(* Logix 5000 AddOnInstructionDefinition export Banner_TL70Pro_Param_v4; software revision 33.00; part 2 of 3 *)
(* tags used below, declared in another part *)
   TL70Pro : Banner_TL70Pro_v4;
   Port_Data : Banner_IOL_Port_v4;
   Port : INT;   // Port Number that device is plugged into.
   Local_Control : DINT;
   Command_Being_Processed : BOOL;
   Update_Archive : BOOL;
   Index_Write_Inprocess : DINT;
   Index_Write_Control : DINT;
   Inprocess_Index : DINT;
   BS_Index : DINT;
   Index_W : DINT;
   W_Index : DINT;
   GT_Index2 : DINT;
   GT_Index1 : DINT;
   LT_Index2 : DINT;
   LT_Index1 : DINT;
(* Banner_TL70Pro_Param_v4, continued *)

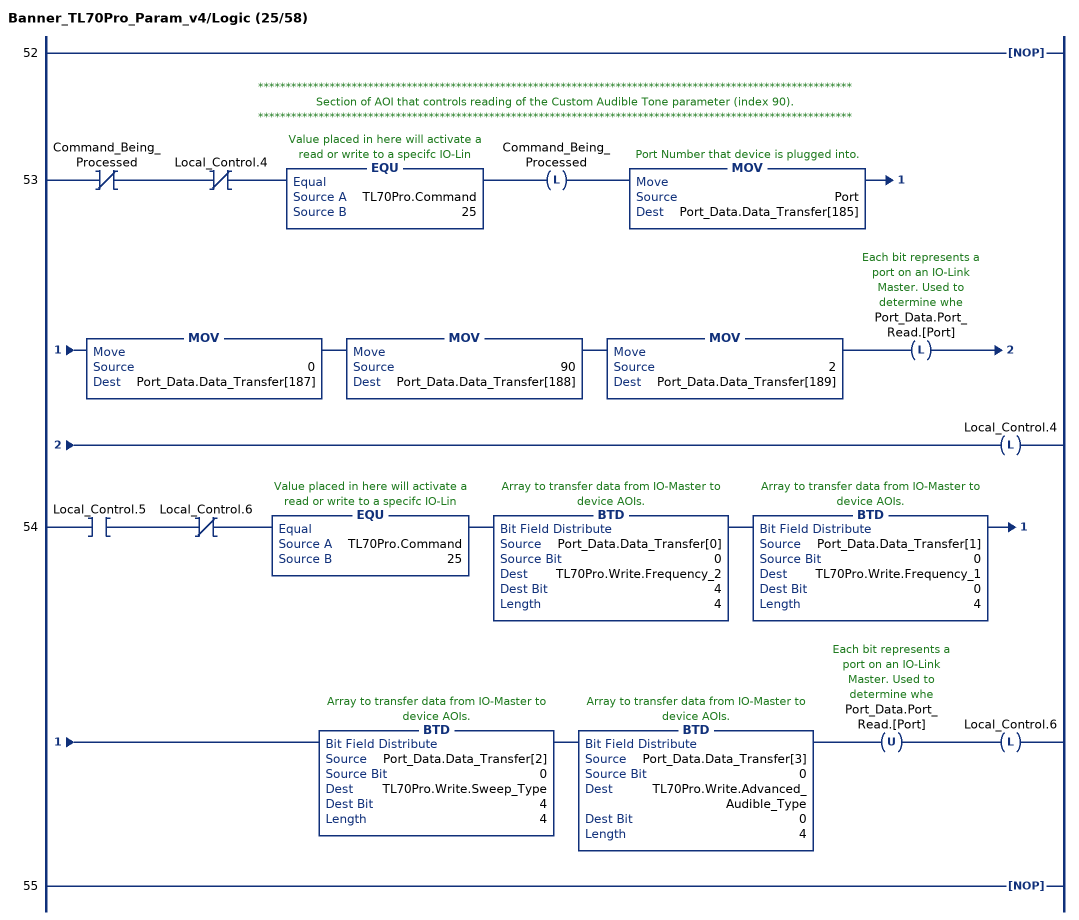
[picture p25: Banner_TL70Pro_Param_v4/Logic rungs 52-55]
   52: NOP();
   // ************************************************************************************************************
   // Section of AOI that controls reading of the Custom Audible Tone parameter (index 90).
   // ************************************************************************************************************
   53: XIO(Command_Being_Processed)XIO(Local_Control.4)EQU(TL70Pro.Command,25)OTL(Command_Being_Processed)MOV(Port,Port_Data.Data_Transfer[185])MOV(0,Port_Data.Data_Transfer[187])MOV(90,Port_Data.Data_Transfer[188])MOV(2,Port_Data.Data_Transfer[189])OTL(Port_Data.Port_Read.[Port])OTL(Local_Control.4);
   54: XIC(Local_Control.5)XIO(Local_Control.6)EQU(TL70Pro.Command,25)BTD(Port_Data.Data_Transfer[0],0,TL70Pro.Write.Frequency_2,4,4)BTD(Port_Data.Data_Transfer[1],0,TL70Pro.Write.Frequency_1,0,4)BTD(Port_Data.Data_Transfer[2],0,TL70Pro.Write.Sweep_Type,4,4)BTD(Port_Data.Data_Transfer[3],0,TL70Pro.Write.Advanced_Audible_Type,0,4)OTU(Port_Data.Port_Read.[Port])OTL(Local_Control.6);
   55: NOP();
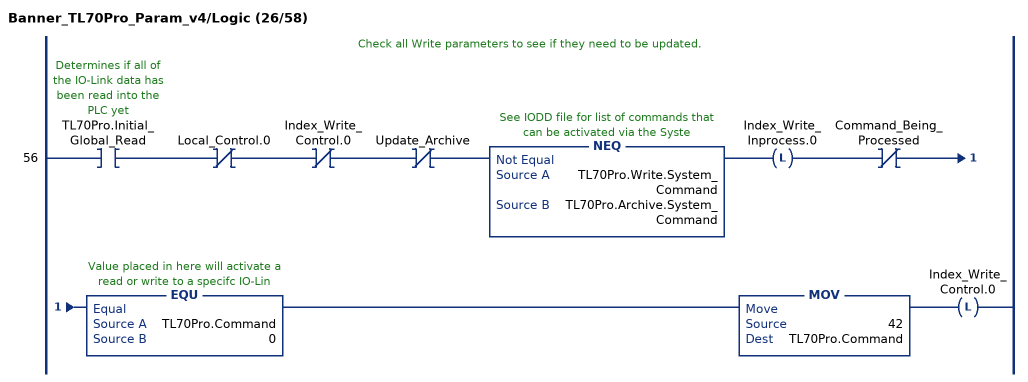
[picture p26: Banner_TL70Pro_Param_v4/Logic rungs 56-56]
   // Check all Write parameters to see if they need to be updated.
   56: XIC(TL70Pro.Initial_Global_Read)XIO(Local_Control.0)XIO(Index_Write_Control.0)XIO(Update_Archive)NEQ(TL70Pro.Write.System_Command,TL70Pro.Archive.System_Command)OTL(Index_Write_Inprocess.0)XIO(Command_Being_Processed)EQU(TL70Pro.Command,0)MOV(42,TL70Pro.Command)OTL(Index_Write_Control.0);
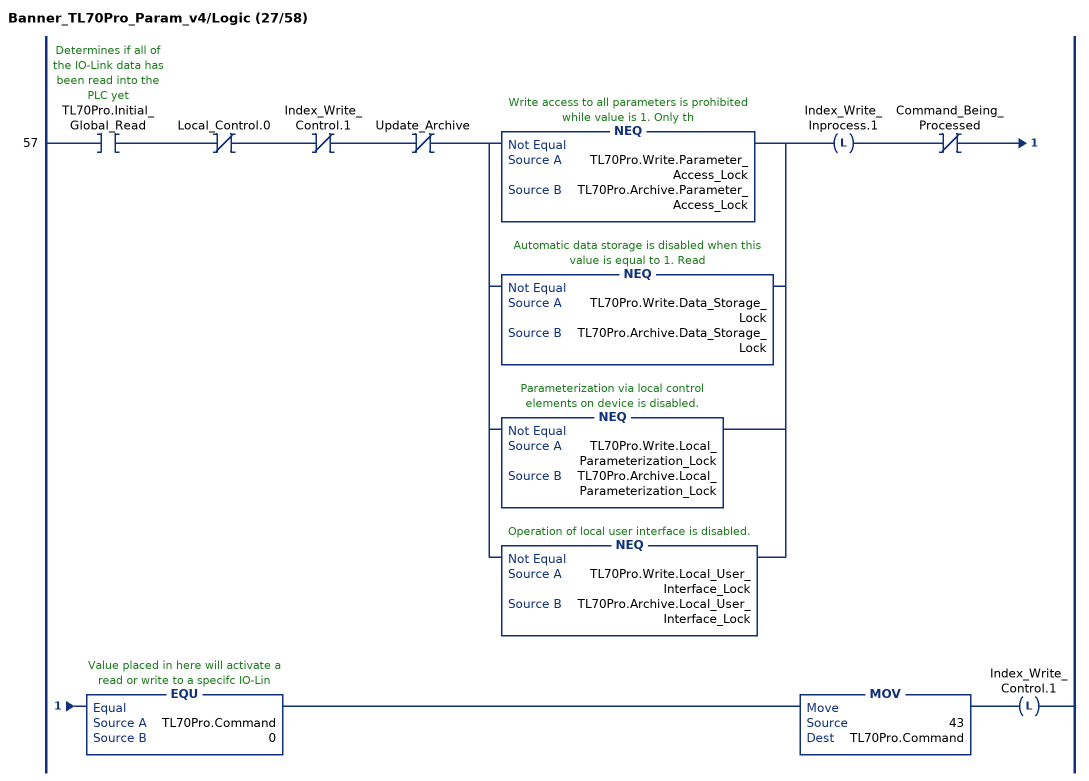
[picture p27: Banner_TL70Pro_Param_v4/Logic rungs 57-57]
   57: XIC(TL70Pro.Initial_Global_Read)XIO(Local_Control.0)XIO(Index_Write_Control.1)XIO(Update_Archive)[NEQ(TL70Pro.Write.Parameter_Access_Lock,TL70Pro.Archive.Parameter_Access_Lock) ,NEQ(TL70Pro.Write.Data_Storage_Lock,TL70Pro.Archive.Data_Storage_Lock) ,NEQ(TL70Pro.Write.Local_Parameterization_Lock,TL70Pro.Archive.Local_Parameterization_Lock) ,NEQ(TL70Pro.Write.Local_User_Interface_Lock,TL70Pro.Archive.Local_User_Interface_Lock) ]OTL(Index_Write_Inprocess.1)XIO(Command_Being_Processed)EQU(TL70Pro.Command,0)MOV(43,TL70Pro.Command)OTL(Index_Write_Control.1);
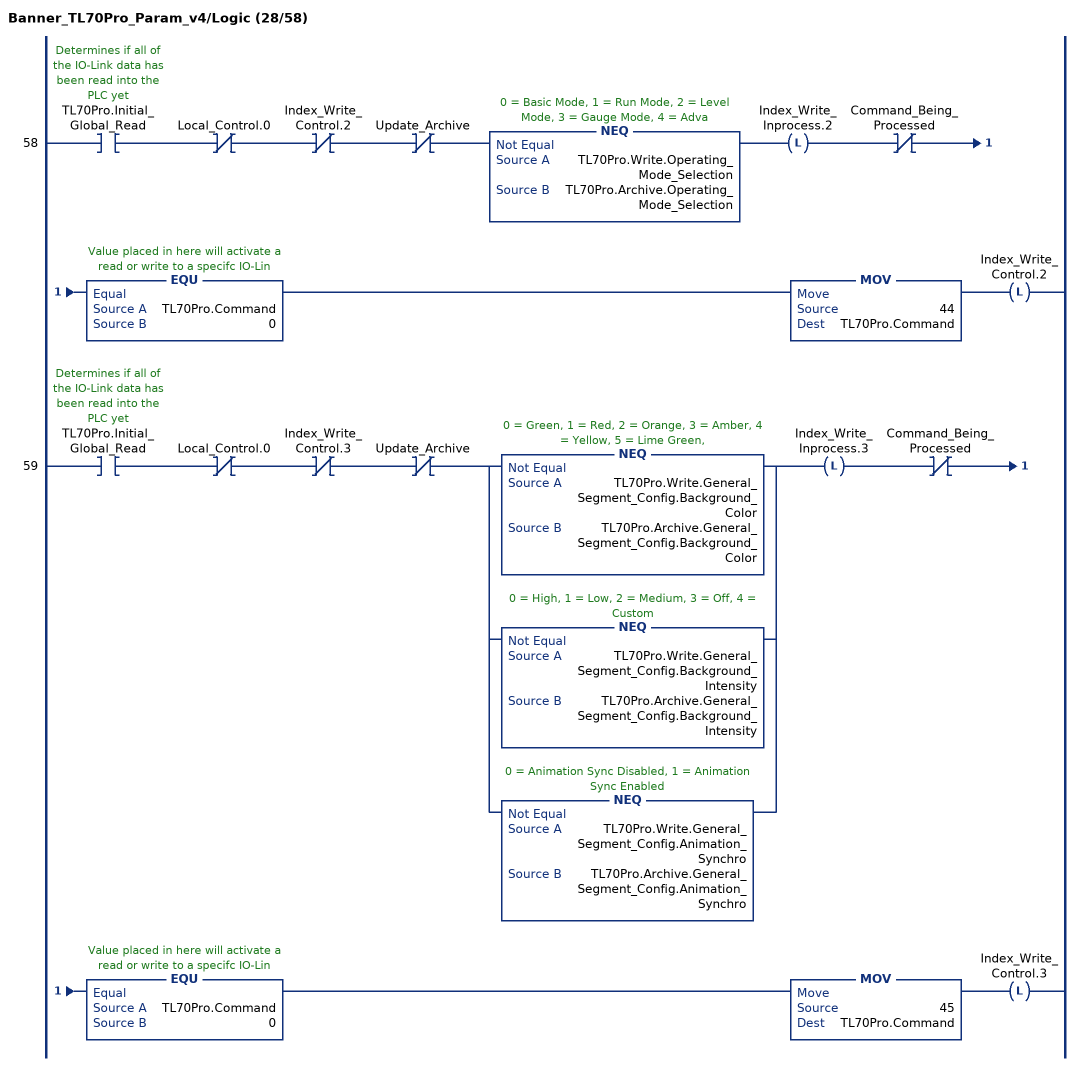
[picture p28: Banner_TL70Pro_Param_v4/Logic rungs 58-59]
   58: XIC(TL70Pro.Initial_Global_Read)XIO(Local_Control.0)XIO(Index_Write_Control.2)XIO(Update_Archive)NEQ(TL70Pro.Write.Operating_Mode_Selection,TL70Pro.Archive.Operating_Mode_Selection)OTL(Index_Write_Inprocess.2)XIO(Command_Being_Processed)EQU(TL70Pro.Command,0)MOV(44,TL70Pro.Command)OTL(Index_Write_Control.2);
   59: XIC(TL70Pro.Initial_Global_Read)XIO(Local_Control.0)XIO(Index_Write_Control.3)XIO(Update_Archive)[NEQ(TL70Pro.Write.General_Segment_Config.Background_Color,TL70Pro.Archive.General_Segment_Config.Background_Color) ,NEQ(TL70Pro.Write.General_Segment_Config.Background_Intensity,TL70Pro.Archive.General_Segment_Config.Background_Intensity) ,NEQ(TL70Pro.Write.General_Segment_Config.Animation_Synchro,TL70Pro.Archive.General_Segment_Config.Animation_Synchro) ]OTL(Index_Write_Inprocess.3)XIO(Command_Being_Processed)EQU(TL70Pro.Command,0)MOV(45,TL70Pro.Command)OTL(Index_Write_Control.3);
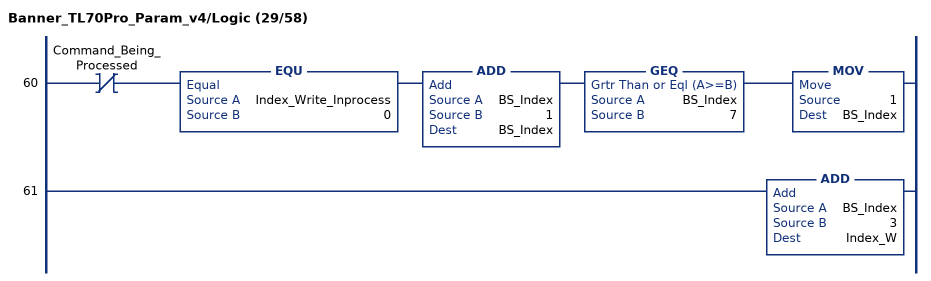
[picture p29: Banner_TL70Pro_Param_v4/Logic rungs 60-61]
   60: XIO(Command_Being_Processed)EQU(Index_Write_Inprocess,0)ADD(BS_Index,1,BS_Index)GEQ(BS_Index,7)MOV(1,BS_Index);
   61: ADD(BS_Index,3,Index_W);
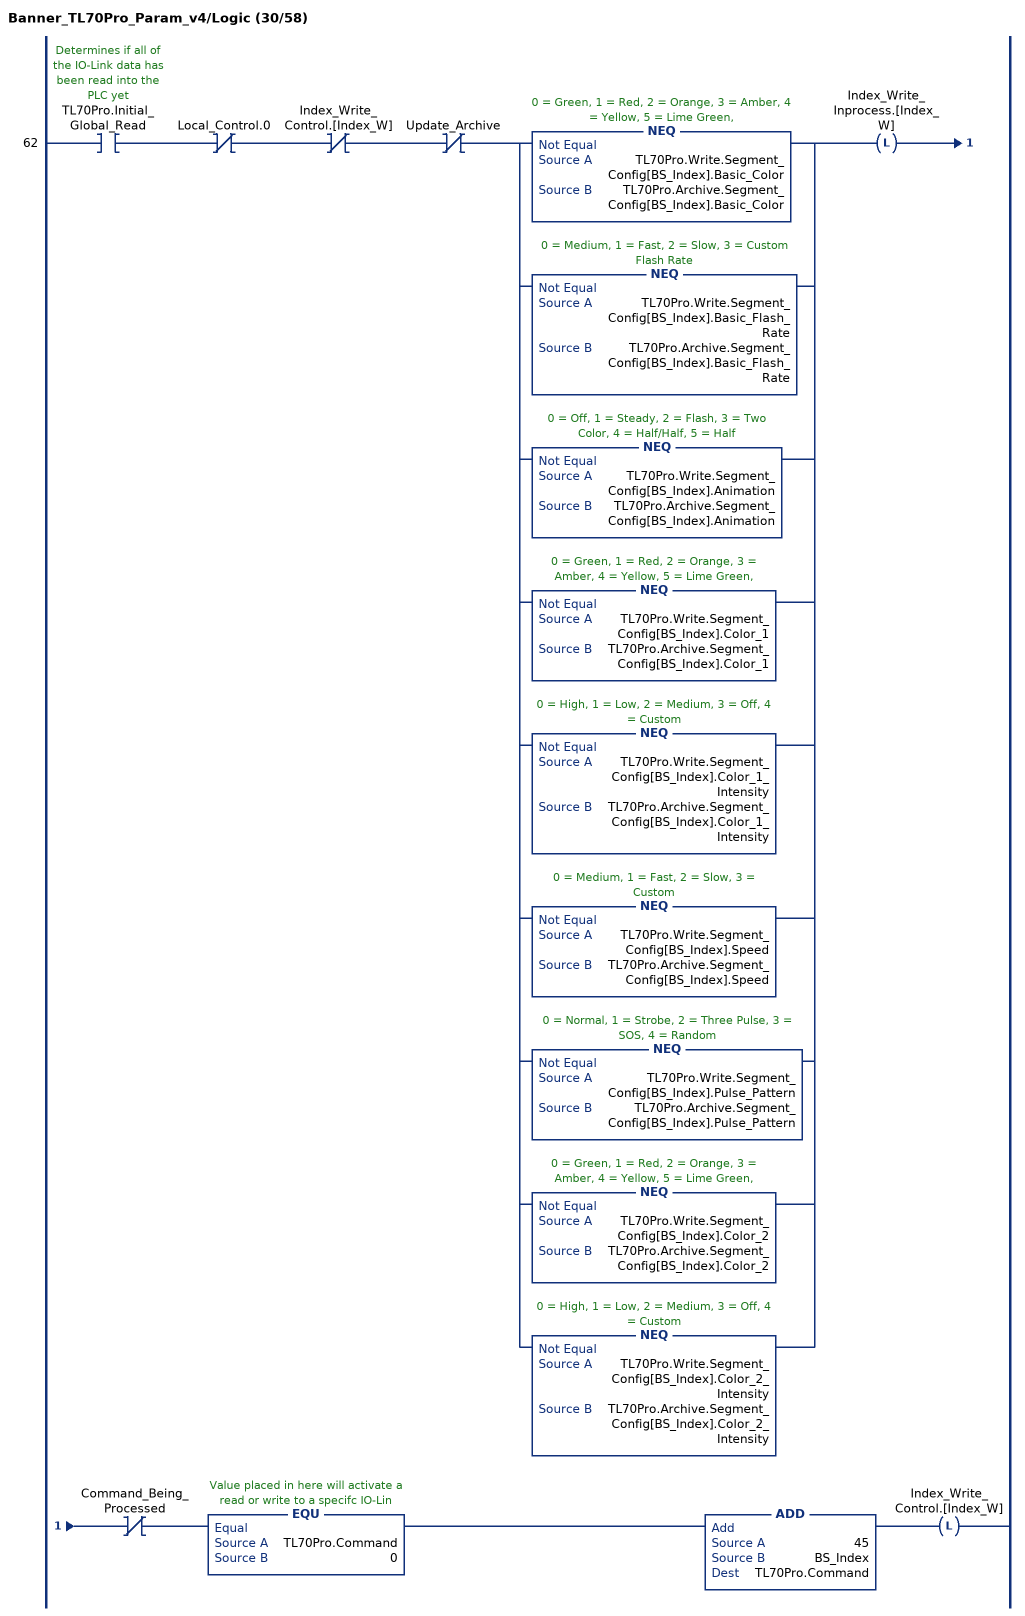
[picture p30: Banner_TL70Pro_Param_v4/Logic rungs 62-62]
   62: XIC(TL70Pro.Initial_Global_Read)XIO(Local_Control.0)XIO(Index_Write_Control.[Index_W])XIO(Update_Archive)[NEQ(TL70Pro.Write.Segment_Config[BS_Index].Basic_Color,TL70Pro.Archive.Segment_Config[BS_Index].Basic_Color) ,NEQ(TL70Pro.Write.Segment_Config[BS_Index].Basic_Flash_Rate,TL70Pro.Archive.Segment_Config[BS_Index].Basic_Flash_Rate) ,NEQ(TL70Pro.Write.Segment_Config[BS_Index].Animation,TL70Pro.Archive.Segment_Config[BS_Index].Animation) ,NEQ(TL70Pro.Write.Segment_Config[BS_Index].Color_1,TL70Pro.Archive.Segment_Config[BS_Index].Color_1) ,NEQ(TL70Pro.Write.Segment_Config[BS_Index].Color_1_Intensity,TL70Pro.Archive.Segment_Config[BS_Index].Color_1_Intensity) ,NEQ(TL70Pro.Write.Segment_Config[BS_Index].Speed,TL70Pro.Archive.Segment_Config[BS_Index].Speed) ,NEQ(TL70Pro.Write.Segment_Config[BS_Index].Pulse_Pattern,TL70Pro.Archive.Segment_Config[BS_Index].Pulse_Pattern) ,NEQ(TL70Pro.Write.Segment_Config[BS_Index].Color_2,TL70Pro.Archive.Segment_Config[BS_Index].Color_2) ,NEQ(TL70Pro.Write.Segment_Config[BS_Index].Color_2_Intensity,TL70Pro.Archive.Segment_Config[BS_Index].Color_2_Intensity) ]OTL(Index_Write_Inprocess.[Index_W])XIO(Command_Being_Processed)EQU(TL70Pro.Command,0)ADD(45,BS_Index,TL70Pro.Command)OTL(Index_Write_Control.[Index_W]);
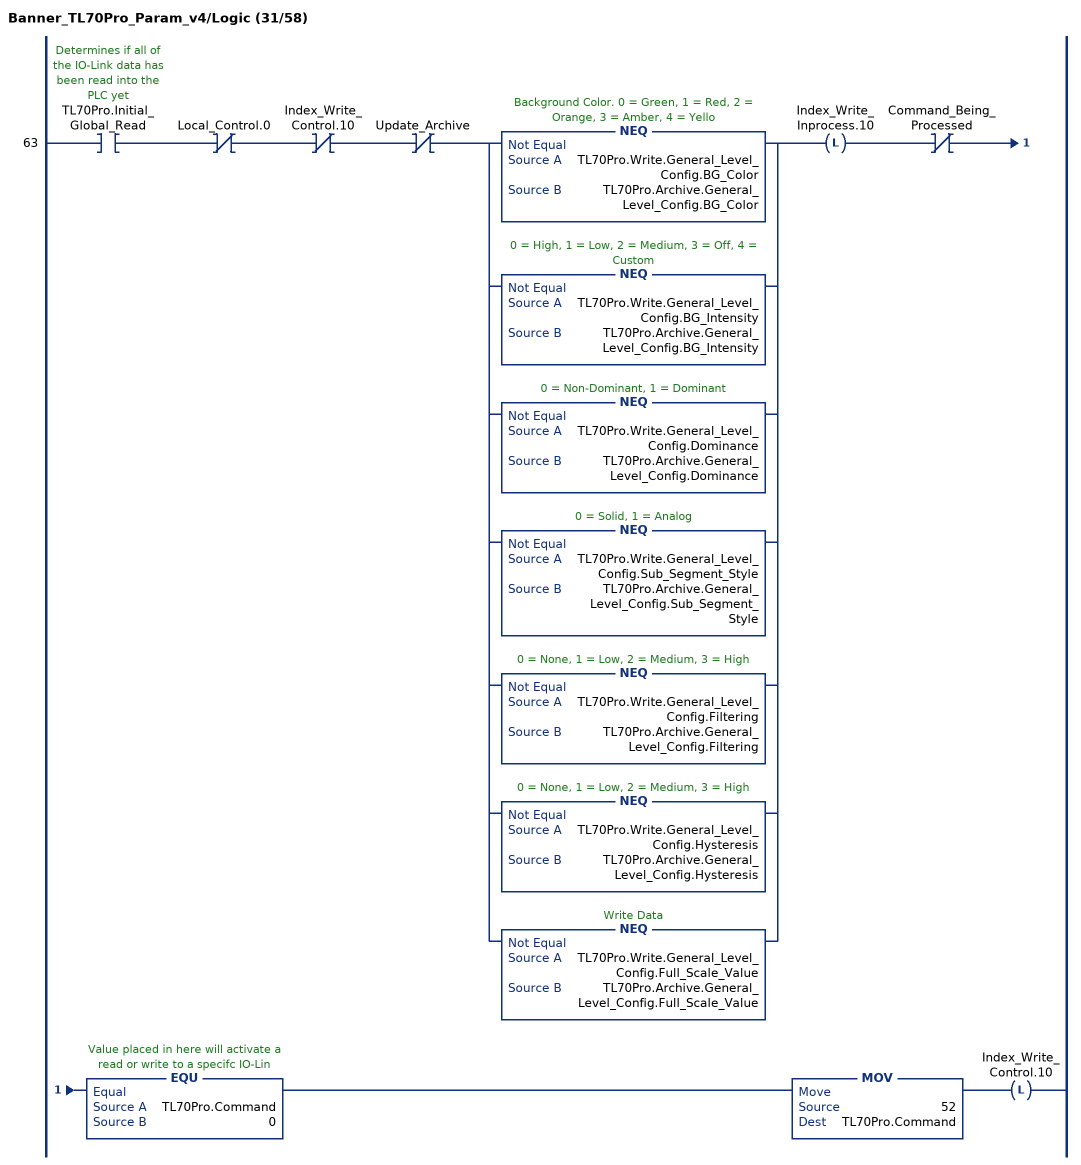
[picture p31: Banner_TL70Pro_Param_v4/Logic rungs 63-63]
   63: XIC(TL70Pro.Initial_Global_Read)XIO(Local_Control.0)XIO(Index_Write_Control.10)XIO(Update_Archive)[NEQ(TL70Pro.Write.General_Level_Config.BG_Color,TL70Pro.Archive.General_Level_Config.BG_Color) ,NEQ(TL70Pro.Write.General_Level_Config.BG_Intensity,TL70Pro.Archive.General_Level_Config.BG_Intensity) ,NEQ(TL70Pro.Write.General_Level_Config.Dominance,TL70Pro.Archive.General_Level_Config.Dominance) ,NEQ(TL70Pro.Write.General_Level_Config.Sub_Segment_Style,TL70Pro.Archive.General_Level_Config.Sub_Segment_Style) ,NEQ(TL70Pro.Write.General_Level_Config.Filtering,TL70Pro.Archive.General_Level_Config.Filtering) ,NEQ(TL70Pro.Write.General_Level_Config.Hysteresis,TL70Pro.Archive.General_Level_Config.Hysteresis) ,NEQ(TL70Pro.Write.General_Level_Config.Full_Scale_Value,TL70Pro.Archive.General_Level_Config.Full_Scale_Value) ]OTL(Index_Write_Inprocess.10)XIO(Command_Being_Processed)EQU(TL70Pro.Command,0)MOV(52,TL70Pro.Command)OTL(Index_Write_Control.10);
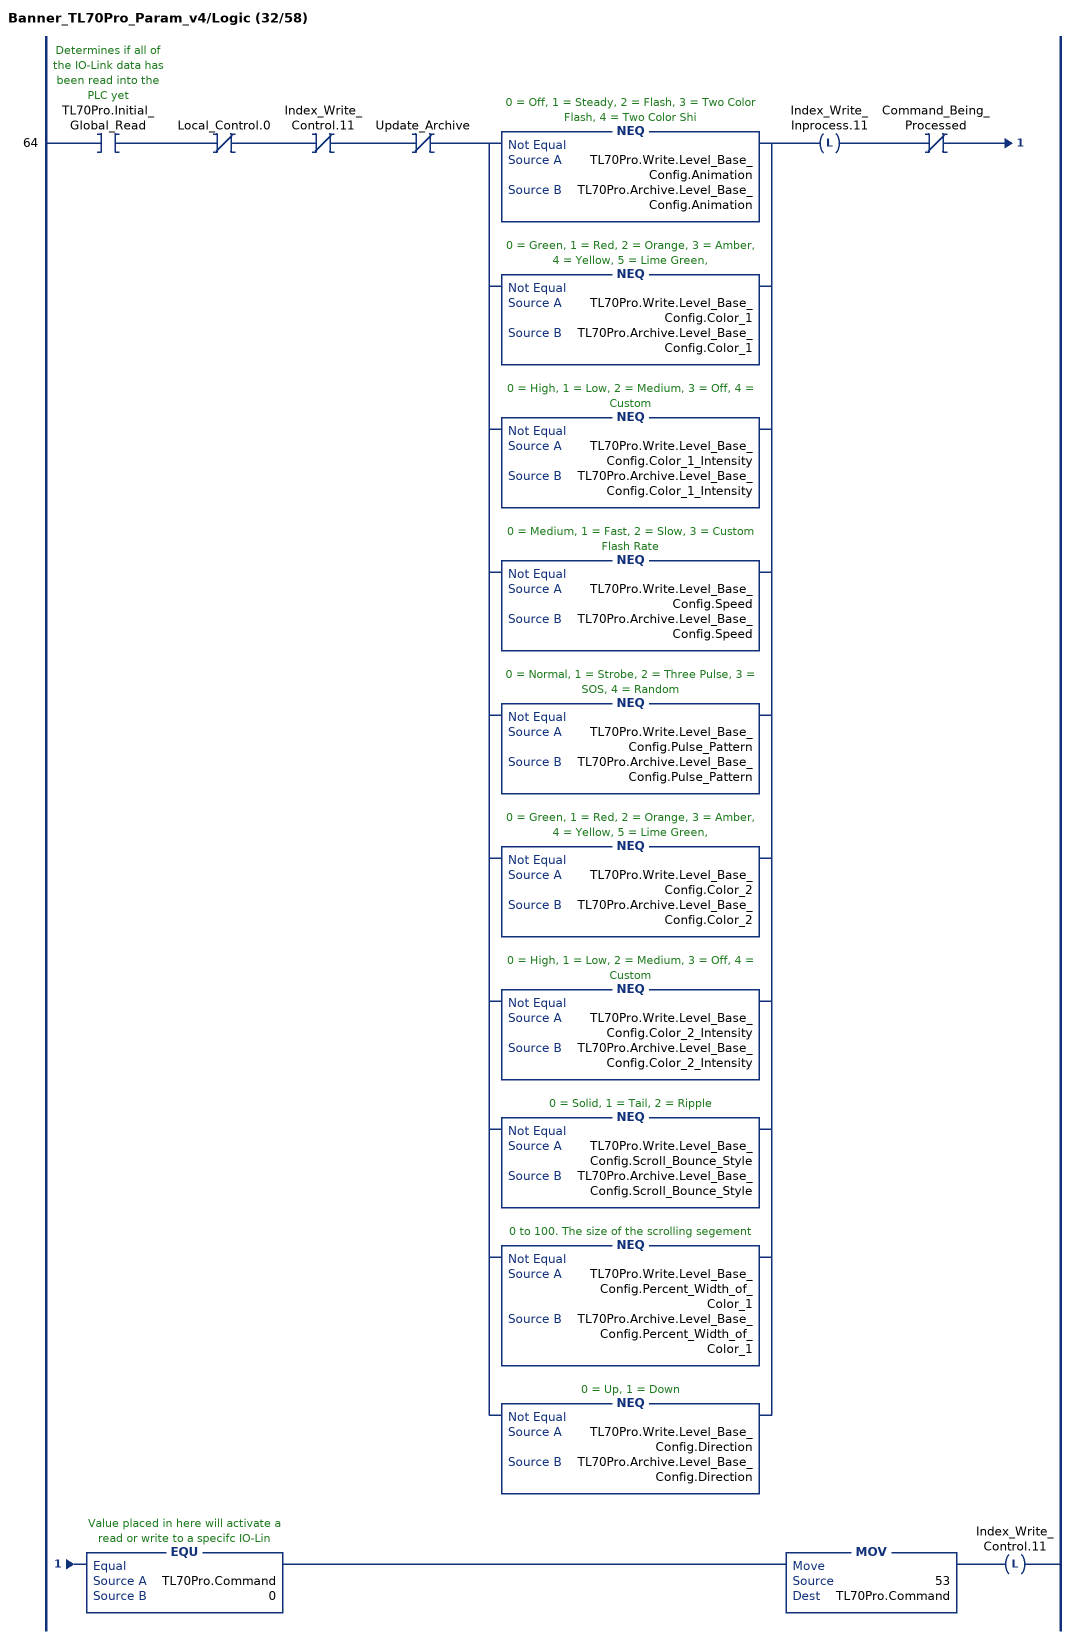
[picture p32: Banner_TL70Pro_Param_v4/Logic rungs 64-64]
   64: XIC(TL70Pro.Initial_Global_Read)XIO(Local_Control.0)XIO(Index_Write_Control.11)XIO(Update_Archive)[NEQ(TL70Pro.Write.Level_Base_Config.Animation,TL70Pro.Archive.Level_Base_Config.Animation) ,NEQ(TL70Pro.Write.Level_Base_Config.Color_1,TL70Pro.Archive.Level_Base_Config.Color_1) ,NEQ(TL70Pro.Write.Level_Base_Config.Color_1_Intensity,TL70Pro.Archive.Level_Base_Config.Color_1_Intensity) ,NEQ(TL70Pro.Write.Level_Base_Config.Speed,TL70Pro.Archive.Level_Base_Config.Speed) ,NEQ(TL70Pro.Write.Level_Base_Config.Pulse_Pattern,TL70Pro.Archive.Level_Base_Config.Pulse_Pattern) ,NEQ(TL70Pro.Write.Level_Base_Config.Color_2,TL70Pro.Archive.Level_Base_Config.Color_2) ,NEQ(TL70Pro.Write.Level_Base_Config.Color_2_Intensity,TL70Pro.Archive.Level_Base_Config.Color_2_Intensity) ,NEQ(TL70Pro.Write.Level_Base_Config.Scroll_Bounce_Style,TL70Pro.Archive.Level_Base_Config.Scroll_Bounce_Style) ,NEQ(TL70Pro.Write.Level_Base_Config.Percent_Width_of_Color_1,TL70Pro.Archive.Level_Base_Config.Percent_Width_of_Color_1) ,NEQ(TL70Pro.Write.Level_Base_Config.Direction,TL70Pro.Archive.Level_Base_Config.Direction) ]OTL(Index_Write_Inprocess.11)XIO(Command_Being_Processed)EQU(TL70Pro.Command,0)MOV(53,TL70Pro.Command)OTL(Index_Write_Control.11);
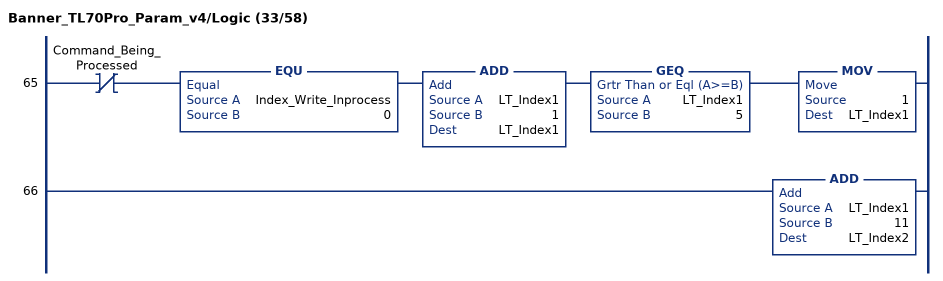
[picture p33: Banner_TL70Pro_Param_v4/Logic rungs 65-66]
   65: XIO(Command_Being_Processed)EQU(Index_Write_Inprocess,0)ADD(LT_Index1,1,LT_Index1)GEQ(LT_Index1,5)MOV(1,LT_Index1);
   66: ADD(LT_Index1,11,LT_Index2);
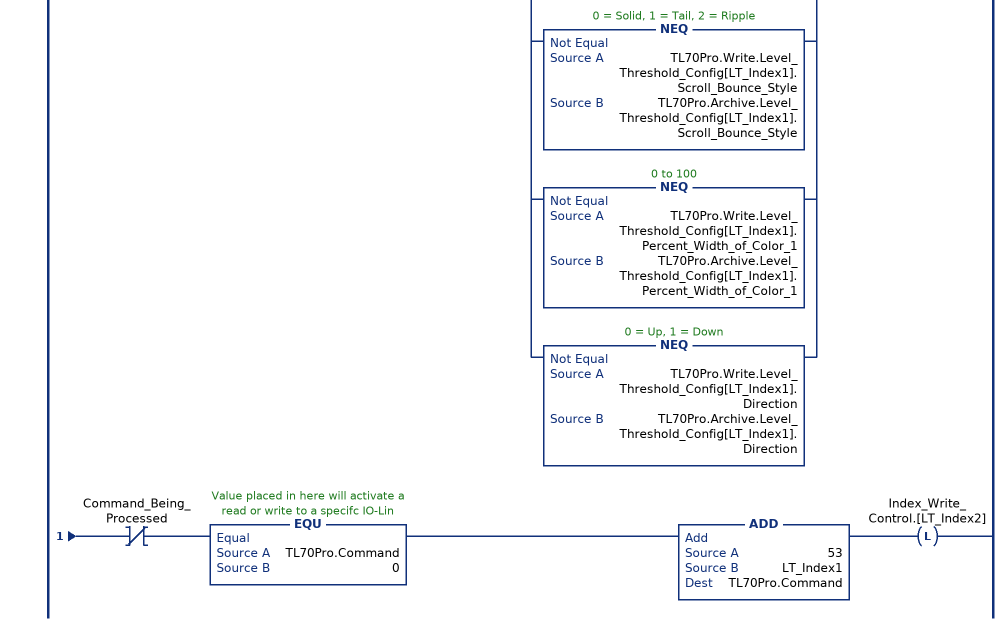
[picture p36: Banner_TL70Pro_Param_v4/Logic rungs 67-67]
   67: XIC(TL70Pro.Initial_Global_Read)XIO(Local_Control.0)XIO(Index_Write_Control.[LT_Index2])XIO(Update_Archive)[NEQ(TL70Pro.Write.Level_Threshold_Config[LT_Index1].Threshold_Enable,TL70Pro.Archive.Level_Threshold_Config[LT_Index1].Threshold_Enable) ,NEQ(TL70Pro.Write.Level_Threshold_Config[LT_Index1].Threshold_Value_Percent,TL70Pro.Archive.Level_Threshold_Config[LT_Index1].Threshold_Value_Percent) ,NEQ(TL70Pro.Write.Level_Threshold_Config[LT_Index1].Threshold_Comparison,TL70Pro.Archive.Level_Threshold_Config[LT_Index1].Threshold_Comparison) ,NEQ(TL70Pro.Write.Level_Threshold_Config[LT_Index1].Threshold_Override,TL70Pro.Archive.Level_Threshold_Config[LT_Index1].Threshold_Override) ,NEQ(TL70Pro.Write.Level_Threshold_Config[LT_Index1].Animation,TL70Pro.Archive.Level_Threshold_Config[LT_Index1].Animation) ,NEQ(TL70Pro.Write.Level_Threshold_Config[LT_Index1].Color_1,TL70Pro.Archive.Level_Threshold_Config[LT_Index1].Color_1) ,NEQ(TL70Pro.Write.Level_Threshold_Config[LT_Index1].Color_1_Intensity,TL70Pro.Archive.Level_Threshold_Config[LT_Index1].Color_1_Intensity) ,NEQ(TL70Pro.Write.Level_Threshold_Config[LT_Index1].Speed,TL70Pro.Archive.Level_Threshold_Config[LT_Index1].Speed) ,NEQ(TL70Pro.Write.Level_Threshold_Config[LT_Index1].Pulse_Pattern,TL70Pro.Archive.Level_Threshold_Config[LT_Index1].Pulse_Pattern) ,NEQ(TL70Pro.Write.Level_Threshold_Config[LT_Index1].Color_2,TL70Pro.Archive.Level_Threshold_Config[LT_Index1].Color_2) ,NEQ(TL70Pro.Write.Level_Threshold_Config[LT_Index1].Color_2_Intensity,TL70Pro.Archive.Level_Threshold_Config[LT_Index1].Color_2_Intensity) ,NEQ(TL70Pro.Write.Level_Threshold_Config[LT_Index1].Scroll_Bounce_Style,TL70Pro.Archive.Level_Threshold_Config[LT_Index1].Scroll_Bounce_Style) ,NEQ(TL70Pro.Write.Level_Threshold_Config[LT_Index1].Percent_Width_of_Color_1,TL70Pro.Archive.Level_Threshold_Config[LT_Index1].Percent_Width_of_Color_1) ,NEQ(TL70Pro.Write.Level_Threshold_Config[LT_Index1].Direction,TL70Pro.Archive.Level_Threshold_Config[LT_Index1].Direction) ]OTL(Index_Write_Inprocess.[LT_Index2])XIO(Command_Being_Processed)EQU(TL70Pro.Command,0)ADD(53,LT_Index1,TL70Pro.Command)OTL(Index_Write_Control.[LT_Index2]);
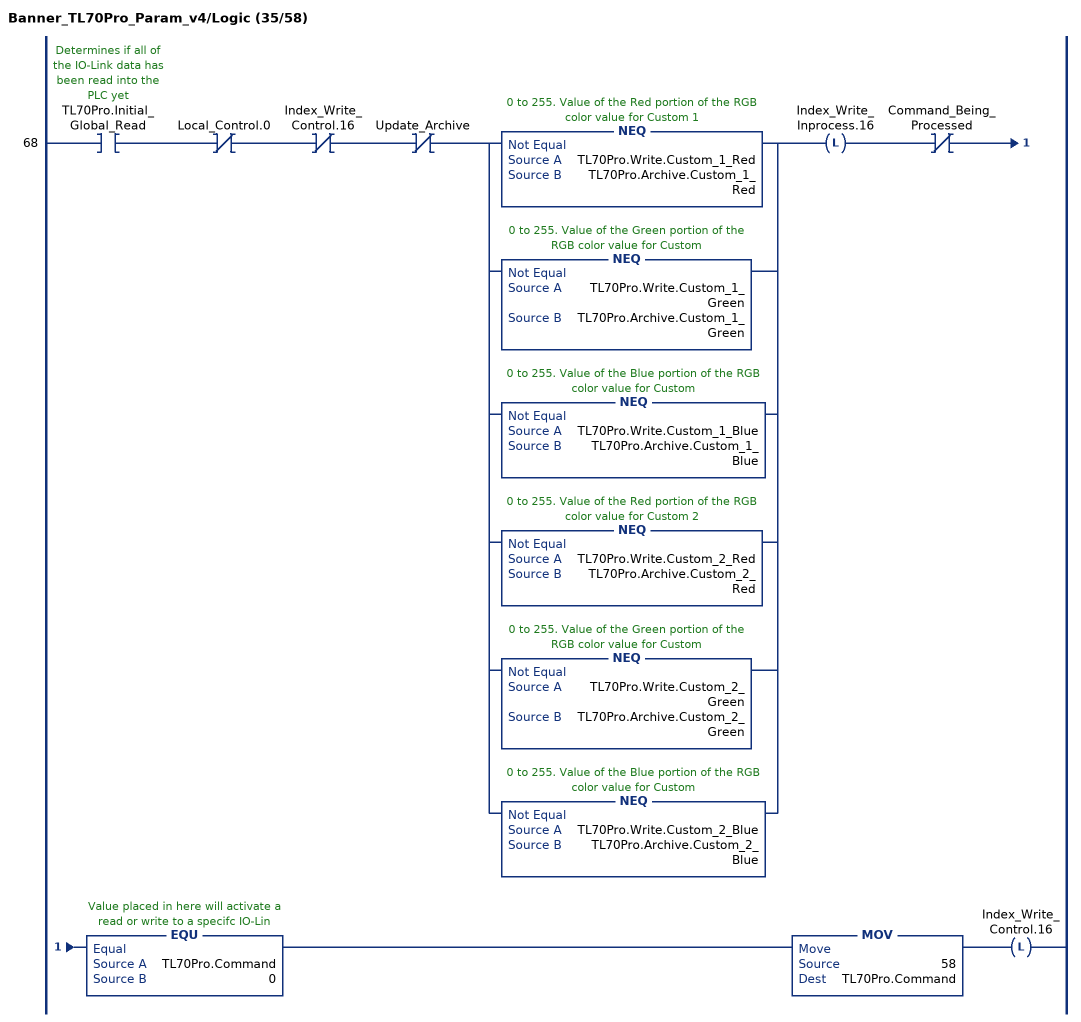
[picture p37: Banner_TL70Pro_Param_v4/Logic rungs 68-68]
   68: XIC(TL70Pro.Initial_Global_Read)XIO(Local_Control.0)XIO(Index_Write_Control.16)XIO(Update_Archive)[NEQ(TL70Pro.Write.Custom_1_Red,TL70Pro.Archive.Custom_1_Red) ,NEQ(TL70Pro.Write.Custom_1_Green,TL70Pro.Archive.Custom_1_Green) ,NEQ(TL70Pro.Write.Custom_1_Blue,TL70Pro.Archive.Custom_1_Blue) ,NEQ(TL70Pro.Write.Custom_2_Red,TL70Pro.Archive.Custom_2_Red) ,NEQ(TL70Pro.Write.Custom_2_Green,TL70Pro.Archive.Custom_2_Green) ,NEQ(TL70Pro.Write.Custom_2_Blue,TL70Pro.Archive.Custom_2_Blue) ]OTL(Index_Write_Inprocess.16)XIO(Command_Being_Processed)EQU(TL70Pro.Command,0)MOV(58,TL70Pro.Command)OTL(Index_Write_Control.16);
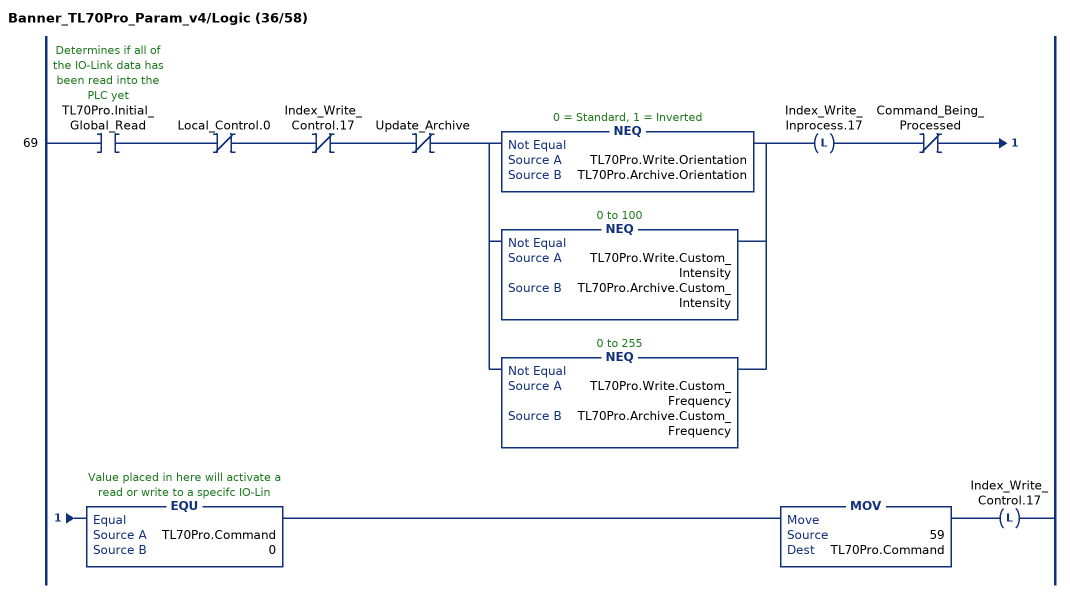
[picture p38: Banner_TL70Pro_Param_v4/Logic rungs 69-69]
   69: XIC(TL70Pro.Initial_Global_Read)XIO(Local_Control.0)XIO(Index_Write_Control.17)XIO(Update_Archive)[NEQ(TL70Pro.Write.Orientation,TL70Pro.Archive.Orientation) ,NEQ(TL70Pro.Write.Custom_Intensity,TL70Pro.Archive.Custom_Intensity) ,NEQ(TL70Pro.Write.Custom_Frequency,TL70Pro.Archive.Custom_Frequency) ]OTL(Index_Write_Inprocess.17)XIO(Command_Being_Processed)EQU(TL70Pro.Command,0)MOV(59,TL70Pro.Command)OTL(Index_Write_Control.17);
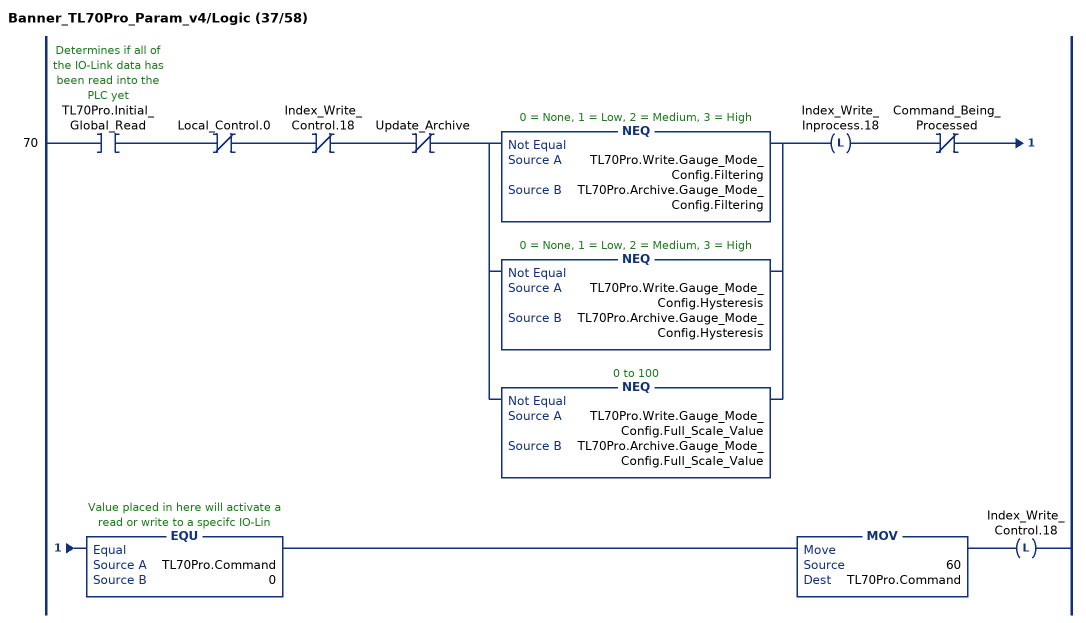
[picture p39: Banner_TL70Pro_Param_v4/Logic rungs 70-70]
   70: XIC(TL70Pro.Initial_Global_Read)XIO(Local_Control.0)XIO(Index_Write_Control.18)XIO(Update_Archive)[NEQ(TL70Pro.Write.Gauge_Mode_Config.Filtering,TL70Pro.Archive.Gauge_Mode_Config.Filtering) ,NEQ(TL70Pro.Write.Gauge_Mode_Config.Hysteresis,TL70Pro.Archive.Gauge_Mode_Config.Hysteresis) ,NEQ(TL70Pro.Write.Gauge_Mode_Config.Full_Scale_Value,TL70Pro.Archive.Gauge_Mode_Config.Full_Scale_Value) ]OTL(Index_Write_Inprocess.18)XIO(Command_Being_Processed)EQU(TL70Pro.Command,0)MOV(60,TL70Pro.Command)OTL(Index_Write_Control.18);
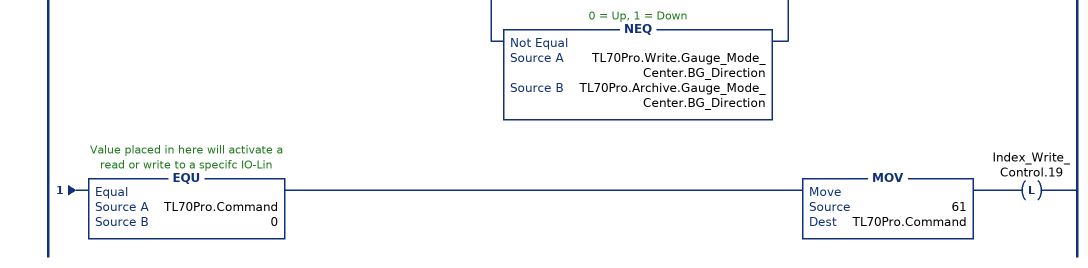
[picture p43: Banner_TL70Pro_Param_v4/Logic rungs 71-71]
   71: XIC(TL70Pro.Initial_Global_Read)XIO(Local_Control.0)XIO(Index_Write_Control.19)XIO(Update_Archive)[NEQ(TL70Pro.Write.Gauge_Mode_Center.Percent_Width_of_Main_Segment,TL70Pro.Archive.Gauge_Mode_Center.Percent_Width_of_Main_Segment) ,NEQ(TL70Pro.Write.Gauge_Mode_Center.Main_Animation,TL70Pro.Archive.Gauge_Mode_Center.Main_Animation) ,NEQ(TL70Pro.Write.Gauge_Mode_Center.Main_Color_1,TL70Pro.Archive.Gauge_Mode_Center.Main_Color_1) ,NEQ(TL70Pro.Write.Gauge_Mode_Center.Main_Color_1_Intensity,TL70Pro.Archive.Gauge_Mode_Center.Main_Color_1_Intensity) ,NEQ(TL70Pro.Write.Gauge_Mode_Center.Main_Speed,TL70Pro.Archive.Gauge_Mode_Center.Main_Speed) ,NEQ(TL70Pro.Write.Gauge_Mode_Center.Main_Pulse_Pattern,TL70Pro.Archive.Gauge_Mode_Center.Main_Pulse_Pattern) ,NEQ(TL70Pro.Write.Gauge_Mode_Center.Main_Color_2,TL70Pro.Archive.Gauge_Mode_Center.Main_Color_2) ,NEQ(TL70Pro.Write.Gauge_Mode_Center.Main_Color_2_Intensity,TL70Pro.Archive.Gauge_Mode_Center.Main_Color_2_Intensity) ,NEQ(TL70Pro.Write.Gauge_Mode_Center.Main_Scroll_Bounce_Style,TL70Pro.Archive.Gauge_Mode_Center.Main_Scroll_Bounce_Style) ,NEQ(TL70Pro.Write.Gauge_Mode_Center.Main_Percent_Width_of_Color_1,TL70Pro.Archive.Gauge_Mode_Center.Main_Percent_Width_of_Color_1) ,NEQ(TL70Pro.Write.Gauge_Mode_Center.Main_Direction,TL70Pro.Archive.Gauge_Mode_Center.Main_Direction) ,NEQ(TL70Pro.Write.Gauge_Mode_Center.BG_Animation,TL70Pro.Archive.Gauge_Mode_Center.BG_Animation) ,NEQ(TL70Pro.Write.Gauge_Mode_Center.BG_Color_1,TL70Pro.Archive.Gauge_Mode_Center.BG_Color_1) ,NEQ(TL70Pro.Write.Gauge_Mode_Center.BG_Color_1_Intensity,TL70Pro.Archive.Gauge_Mode_Center.BG_Color_1_Intensity) ,NEQ(TL70Pro.Write.Gauge_Mode_Center.BG_Speed,TL70Pro.Archive.Gauge_Mode_Center.BG_Speed) ,NEQ(TL70Pro.Write.Gauge_Mode_Center.BG_Pulse_Pattern,TL70Pro.Archive.Gauge_Mode_Center.BG_Pulse_Pattern) ,NEQ(TL70Pro.Write.Gauge_Mode_Center.BG_Color_2,TL70Pro.Archive.Gauge_Mode_Center.BG_Color_2) ,NEQ(TL70Pro.Write.Gauge_Mode_Center.BG_Color_2_Intensity,TL70Pro.Archive.Gauge_Mode_Center.BG_Color_2_Intensity) ,NEQ(TL70Pro.Write.Gauge_Mode_Center.BG_Scroll_Bounce_Style,TL70Pro.Archive.Gauge_Mode_Center.BG_Scroll_Bounce_Style) ,NEQ(TL70Pro.Write.Gauge_Mode_Center.BG_Percent_Width_of_Color_1,TL70Pro.Archive.Gauge_Mode_Center.BG_Percent_Width_of_Color_1) ,NEQ(TL70Pro.Write.Gauge_Mode_Center.BG_Direction,TL70Pro.Archive.Gauge_Mode_Center.BG_Direction) ]OTL(Index_Write_Inprocess.19)XIO(Command_Being_Processed)EQU(TL70Pro.Command,0)MOV(61,TL70Pro.Command)OTL(Index_Write_Control.19);
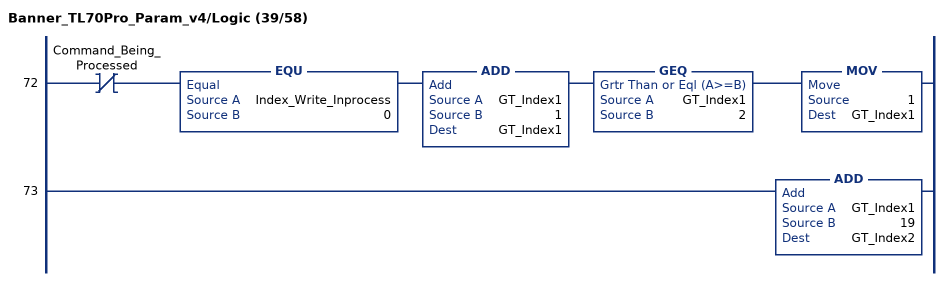
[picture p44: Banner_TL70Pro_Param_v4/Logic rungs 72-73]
   72: XIO(Command_Being_Processed)EQU(Index_Write_Inprocess,0)ADD(GT_Index1,1,GT_Index1)GEQ(GT_Index1,2)MOV(1,GT_Index1);
   73: ADD(GT_Index1,19,GT_Index2);
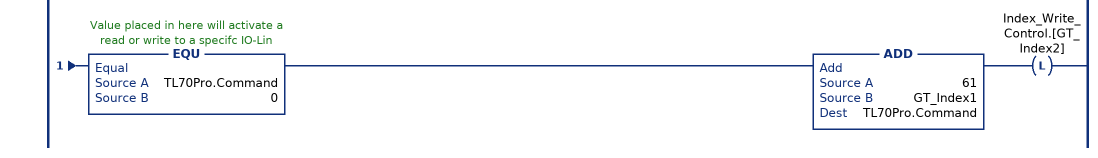
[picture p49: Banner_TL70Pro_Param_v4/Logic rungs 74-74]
   74: XIC(TL70Pro.Initial_Global_Read)XIO(Local_Control.0)XIO(Index_Write_Control.[GT_Index2])XIO(Update_Archive)[NEQ(TL70Pro.Write.Gauge_Mode_Threshold[GT_Index1].Threshold_Enable,TL70Pro.Archive.Gauge_Mode_Threshold[GT_Index1].Threshold_Enable) ,NEQ(TL70Pro.Write.Gauge_Mode_Threshold[GT_Index1].Threshold_Value,TL70Pro.Archive.Gauge_Mode_Threshold[GT_Index1].Threshold_Value) ,NEQ(TL70Pro.Write.Gauge_Mode_Threshold[GT_Index1].Threshold_Comparison,TL70Pro.Archive.Gauge_Mode_Threshold[GT_Index1].Threshold_Comparison) ,NEQ(TL70Pro.Write.Gauge_Mode_Threshold[GT_Index1].Percent_Width_of_Main_Segment,TL70Pro.Archive.Gauge_Mode_Threshold[GT_Index1].Percent_Width_of_Main_Segment) ,NEQ(TL70Pro.Write.Gauge_Mode_Threshold[GT_Index1].Main_Animation,TL70Pro.Archive.Gauge_Mode_Threshold[GT_Index1].Main_Animation) ,NEQ(TL70Pro.Write.Gauge_Mode_Threshold[GT_Index1].Main_Color_1,TL70Pro.Archive.Gauge_Mode_Threshold[GT_Index1].Main_Color_1) ,NEQ(TL70Pro.Write.Gauge_Mode_Threshold[GT_Index1].Main_Color_1_Intensity,TL70Pro.Archive.Gauge_Mode_Threshold[GT_Index1].Main_Color_1_Intensity) ,NEQ(TL70Pro.Write.Gauge_Mode_Threshold[GT_Index1].Main_Speed,TL70Pro.Archive.Gauge_Mode_Threshold[GT_Index1].Main_Speed) ,NEQ(TL70Pro.Write.Gauge_Mode_Threshold[GT_Index1].Main_Pulse_Pattern,TL70Pro.Archive.Gauge_Mode_Threshold[GT_Index1].Main_Pulse_Pattern) ,NEQ(TL70Pro.Write.Gauge_Mode_Threshold[GT_Index1].Main_Color_2,TL70Pro.Archive.Gauge_Mode_Threshold[GT_Index1].Main_Color_2) ,NEQ(TL70Pro.Write.Gauge_Mode_Threshold[GT_Index1].Main_Color_2_Intensity,TL70Pro.Archive.Gauge_Mode_Threshold[GT_Index1].Main_Color_2_Intensity) ,NEQ(TL70Pro.Write.Gauge_Mode_Threshold[GT_Index1].Main_Scroll_Bounce_Style,TL70Pro.Archive.Gauge_Mode_Threshold[GT_Index1].Main_Scroll_Bounce_Style) ,NEQ(TL70Pro.Write.Gauge_Mode_Threshold[GT_Index1].Main_Percent_Width_of_Color_1,TL70Pro.Archive.Gauge_Mode_Threshold[GT_Index1].Main_Percent_Width_of_Color_1) ,NEQ(TL70Pro.Write.Gauge_Mode_Threshold[GT_Index1].Main_Direction,TL70Pro.Archive.Gauge_Mode_Threshold[GT_Index1].Main_Direction) ,NEQ(TL70Pro.Write.Gauge_Mode_Threshold[GT_Index1].BG_Animation,TL70Pro.Archive.Gauge_Mode_Threshold[GT_Index1].BG_Animation) ,NEQ(TL70Pro.Write.Gauge_Mode_Threshold[GT_Index1].BG_Color_1,TL70Pro.Archive.Gauge_Mode_Threshold[GT_Index1].BG_Color_1) ,NEQ(TL70Pro.Write.Gauge_Mode_Threshold[GT_Index1].BG_Color_1_Intensity,TL70Pro.Archive.Gauge_Mode_Threshold[GT_Index1].BG_Color_1_Intensity) ,NEQ(TL70Pro.Write.Gauge_Mode_Threshold[GT_Index1].BG_Speed,TL70Pro.Archive.Gauge_Mode_Threshold[GT_Index1].BG_Speed) ,NEQ(TL70Pro.Write.Gauge_Mode_Threshold[GT_Index1].BG_Pulse_Pattern,TL70Pro.Archive.Gauge_Mode_Threshold[GT_Index1].BG_Pulse_Pattern) ,NEQ(TL70Pro.Write.Gauge_Mode_Threshold[GT_Index1].BG_Color_2,TL70Pro.Archive.Gauge_Mode_Threshold[GT_Index1].BG_Color_2) ,NEQ(TL70Pro.Write.Gauge_Mode_Threshold[GT_Index1].BG_Color_2_Intensity,TL70Pro.Archive.Gauge_Mode_Threshold[GT_Index1].BG_Color_2_Intensity) ,NEQ(TL70Pro.Write.Gauge_Mode_Threshold[GT_Index1].BG_Scroll_Bounce_Style,TL70Pro.Archive.Gauge_Mode_Threshold[GT_Index1].BG_Scroll_Bounce_Style) ,NEQ(TL70Pro.Write.Gauge_Mode_Threshold[GT_Index1].BG_Percent_Width_of_Color_1,TL70Pro.Archive.Gauge_Mode_Threshold[GT_Index1].BG_Percent_Width_of_Color_1) ,NEQ(TL70Pro.Write.Gauge_Mode_Threshold[GT_Index1].BG_Direction,TL70Pro.Archive.Gauge_Mode_Threshold[GT_Index1].BG_Direction) ]OTL(Index_Write_Inprocess.[GT_Index2])XIO(Command_Being_Processed)EQU(TL70Pro.Command,0)ADD(61,GT_Index1,TL70Pro.Command)OTL(Index_Write_Control.[GT_Index2]);
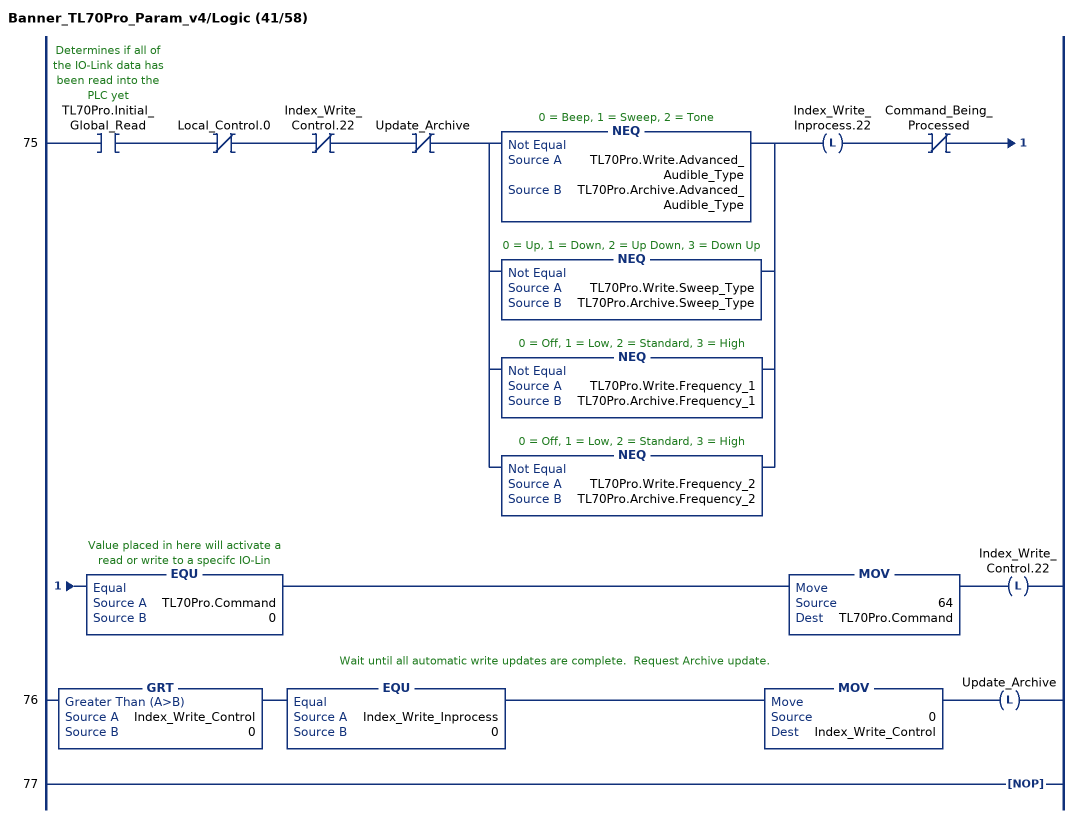
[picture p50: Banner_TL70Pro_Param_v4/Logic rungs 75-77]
   75: XIC(TL70Pro.Initial_Global_Read)XIO(Local_Control.0)XIO(Index_Write_Control.22)XIO(Update_Archive)[NEQ(TL70Pro.Write.Advanced_Audible_Type,TL70Pro.Archive.Advanced_Audible_Type) ,NEQ(TL70Pro.Write.Sweep_Type,TL70Pro.Archive.Sweep_Type) ,NEQ(TL70Pro.Write.Frequency_1,TL70Pro.Archive.Frequency_1) ,NEQ(TL70Pro.Write.Frequency_2,TL70Pro.Archive.Frequency_2) ]OTL(Index_Write_Inprocess.22)XIO(Command_Being_Processed)EQU(TL70Pro.Command,0)MOV(64,TL70Pro.Command)OTL(Index_Write_Control.22);
   // Wait until all automatic write updates are complete.  Request Archive update.
   76: GRT(Index_Write_Control,0)EQU(Index_Write_Inprocess,0)MOV(0,Index_Write_Control)OTL(Update_Archive);
   77: NOP();
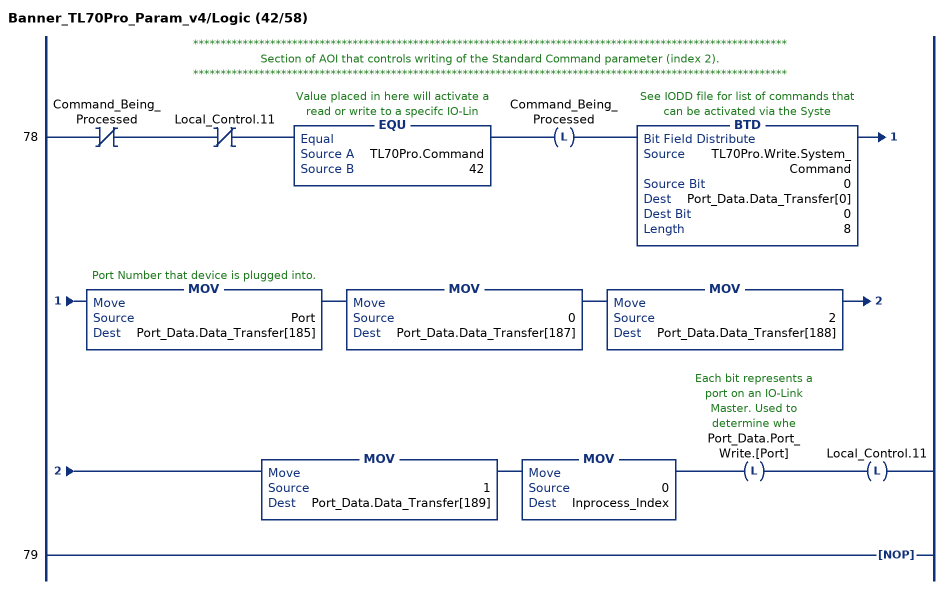
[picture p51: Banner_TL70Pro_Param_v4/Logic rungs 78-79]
   // ************************************************************************************************************
   // Section of AOI that controls writing of the Standard Command parameter (index 2).
   // ************************************************************************************************************
   78: XIO(Command_Being_Processed)XIO(Local_Control.11)EQU(TL70Pro.Command,42)OTL(Command_Being_Processed)BTD(TL70Pro.Write.System_Command,0,Port_Data.Data_Transfer[0],0,8)MOV(Port,Port_Data.Data_Transfer[185])MOV(0,Port_Data.Data_Transfer[187])MOV(2,Port_Data.Data_Transfer[188])MOV(1,Port_Data.Data_Transfer[189])MOV(0,Inprocess_Index)OTL(Port_Data.Port_Write.[Port])OTL(Local_Control.11);
   79: NOP();
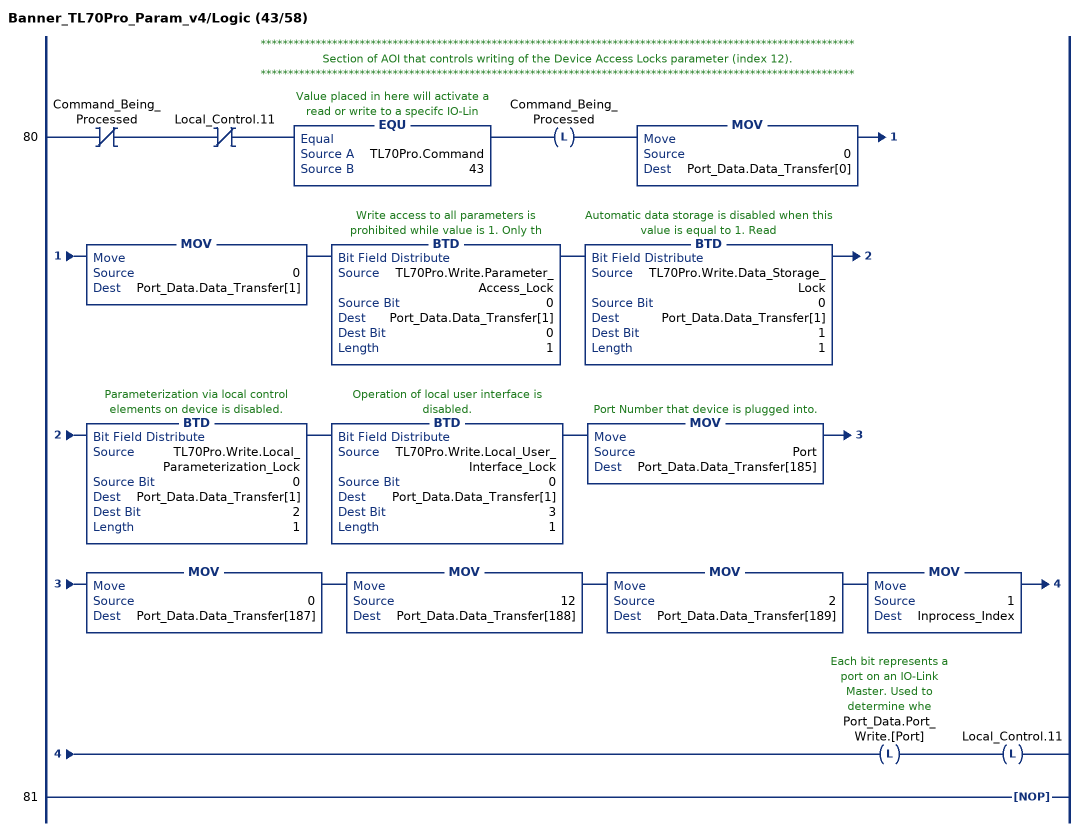
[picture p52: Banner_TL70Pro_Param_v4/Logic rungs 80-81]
   // ************************************************************************************************************
   // Section of AOI that controls writing of the Device Access Locks parameter (index 12).
   // ************************************************************************************************************
   80: XIO(Command_Being_Processed)XIO(Local_Control.11)EQU(TL70Pro.Command,43)OTL(Command_Being_Processed)MOV(0,Port_Data.Data_Transfer[0])MOV(0,Port_Data.Data_Transfer[1])BTD(TL70Pro.Write.Parameter_Access_Lock,0,Port_Data.Data_Transfer[1],0,1)BTD(TL70Pro.Write.Data_Storage_Lock,0,Port_Data.Data_Transfer[1],1,1)BTD(TL70Pro.Write.Local_Parameterization_Lock,0,Port_Data.Data_Transfer[1],2,1)BTD(TL70Pro.Write.Local_User_Interface_Lock,0,Port_Data.Data_Transfer[1],3,1)MOV(Port,Port_Data.Data_Transfer[185])MOV(0,Port_Data.Data_Transfer[187])MOV(12,Port_Data.Data_Transfer[188])MOV(2,Port_Data.Data_Transfer[189])MOV(1,Inprocess_Index)OTL(Port_Data.Port_Write.[Port])OTL(Local_Control.11);
   81: NOP();
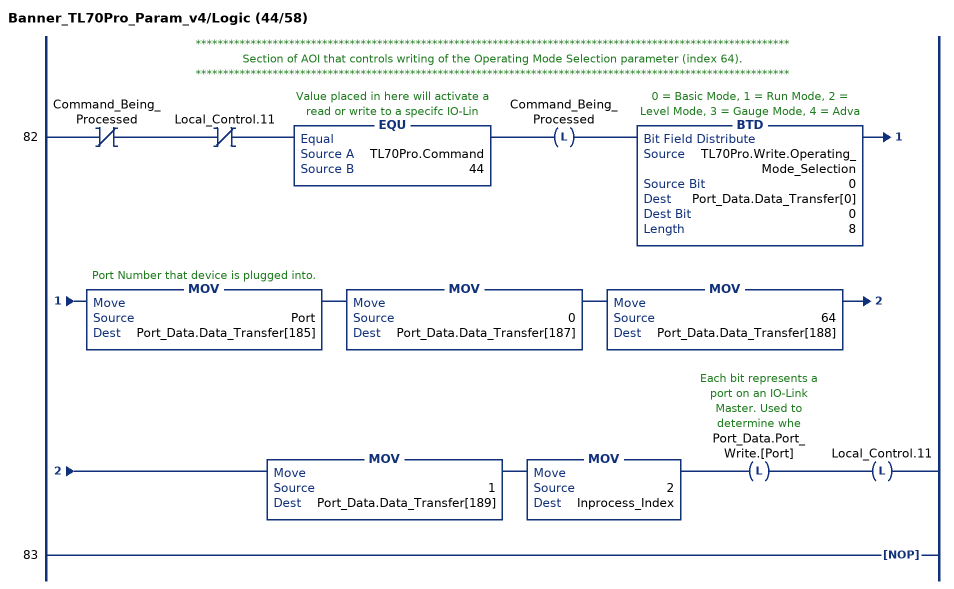
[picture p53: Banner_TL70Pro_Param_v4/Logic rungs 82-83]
   // ************************************************************************************************************
   // Section of AOI that controls writing of the Operating Mode Selection parameter (index 64).
   // ************************************************************************************************************
   82: XIO(Command_Being_Processed)XIO(Local_Control.11)EQU(TL70Pro.Command,44)OTL(Command_Being_Processed)BTD(TL70Pro.Write.Operating_Mode_Selection,0,Port_Data.Data_Transfer[0],0,8)MOV(Port,Port_Data.Data_Transfer[185])MOV(0,Port_Data.Data_Transfer[187])MOV(64,Port_Data.Data_Transfer[188])MOV(1,Port_Data.Data_Transfer[189])MOV(2,Inprocess_Index)OTL(Port_Data.Port_Write.[Port])OTL(Local_Control.11);
   83: NOP();
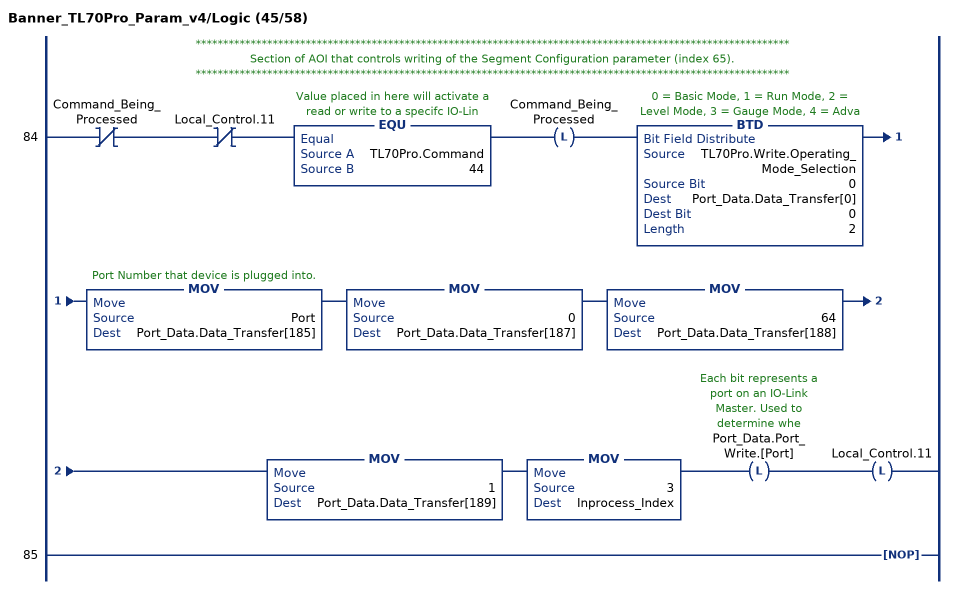
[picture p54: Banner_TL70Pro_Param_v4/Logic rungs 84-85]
   // ************************************************************************************************************
   // Section of AOI that controls writing of the Segment Configuration parameter (index 65).
   // ************************************************************************************************************
   84: XIO(Command_Being_Processed)XIO(Local_Control.11)EQU(TL70Pro.Command,44)OTL(Command_Being_Processed)BTD(TL70Pro.Write.Operating_Mode_Selection,0,Port_Data.Data_Transfer[0],0,2)MOV(Port,Port_Data.Data_Transfer[185])MOV(0,Port_Data.Data_Transfer[187])MOV(64,Port_Data.Data_Transfer[188])MOV(1,Port_Data.Data_Transfer[189])MOV(3,Inprocess_Index)OTL(Port_Data.Port_Write.[Port])OTL(Local_Control.11);
   85: NOP();
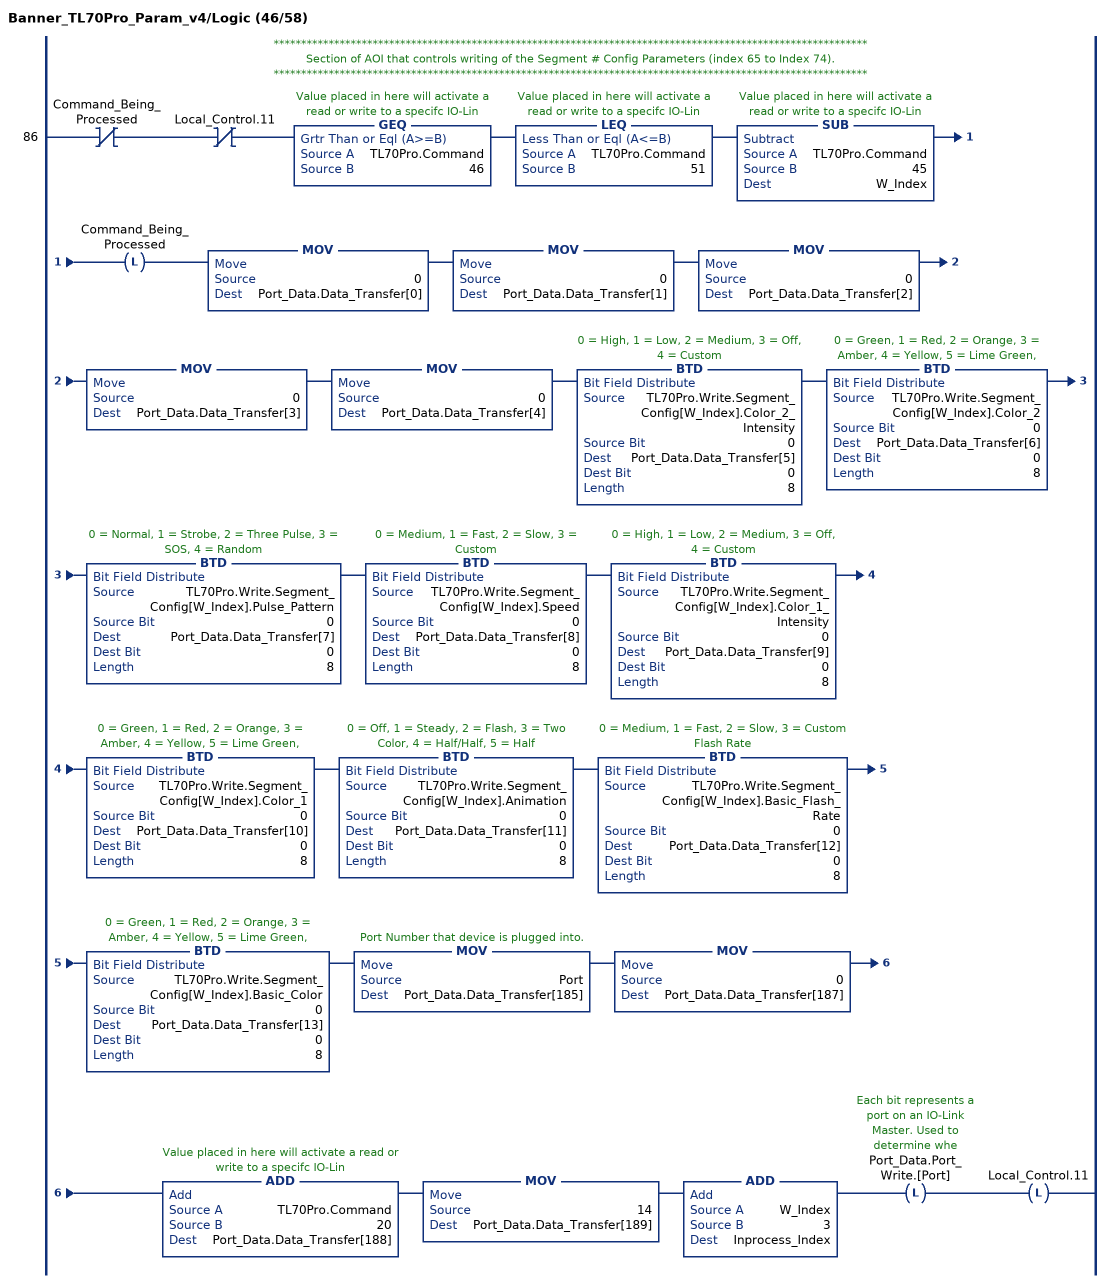
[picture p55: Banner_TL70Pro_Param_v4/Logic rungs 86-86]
   // ************************************************************************************************************
   // Section of AOI that controls writing of the Segment # Config Parameters (index 65 to Index 74).
   // ************************************************************************************************************
   86: XIO(Command_Being_Processed)XIO(Local_Control.11)GEQ(TL70Pro.Command,46)LEQ(TL70Pro.Command,51)SUB(TL70Pro.Command,45,W_Index)OTL(Command_Being_Processed)MOV(0,Port_Data.Data_Transfer[0])MOV(0,Port_Data.Data_Transfer[1])MOV(0,Port_Data.Data_Transfer[2])MOV(0,Port_Data.Data_Transfer[3])MOV(0,Port_Data.Data_Transfer[4])BTD(TL70Pro.Write.Segment_Config[W_Index].Color_2_Intensity,0,Port_Data.Data_Transfer[5],0,8)BTD(TL70Pro.Write.Segment_Config[W_Index].Color_2,0,Port_Data.Data_Transfer[6],0,8)BTD(TL70Pro.Write.Segment_Config[W_Index].Pulse_Pattern,0,Port_Data.Data_Transfer[7],0,8)BTD(TL70Pro.Write.Segment_Config[W_Index].Speed,0,Port_Data.Data_Transfer[8],0,8)BTD(TL70Pro.Write.Segment_Config[W_Index].Color_1_Intensity,0,Port_Data.Data_Transfer[9],0,8)BTD(TL70Pro.Write.Segment_Config[W_Index].Color_1,0,Port_Data.Data_Transfer[10],0,8)BTD(TL70Pro.Write.Segment_Config[W_Index].Animation,0,Port_Data.Data_Transfer[11],0,8)BTD(TL70Pro.Write.Segment_Config[W_Index].Basic_Flash_Rate,0,Port_Data.Data_Transfer[12],0,8)BTD(TL70Pro.Write.Segment_Config[W_Index].Basic_Color,0,Port_Data.Data_Transfer[13],0,8)MOV(Port,Port_Data.Data_Transfer[185])MOV(0,Port_Data.Data_Transfer[187])ADD(TL70Pro.Command,20,Port_Data.Data_Transfer[188])MOV(14,Port_Data.Data_Transfer[189])ADD(W_Index,3,Inprocess_Index)OTL(Port_Data.Port_Write.[Port])OTL(Local_Control.11);
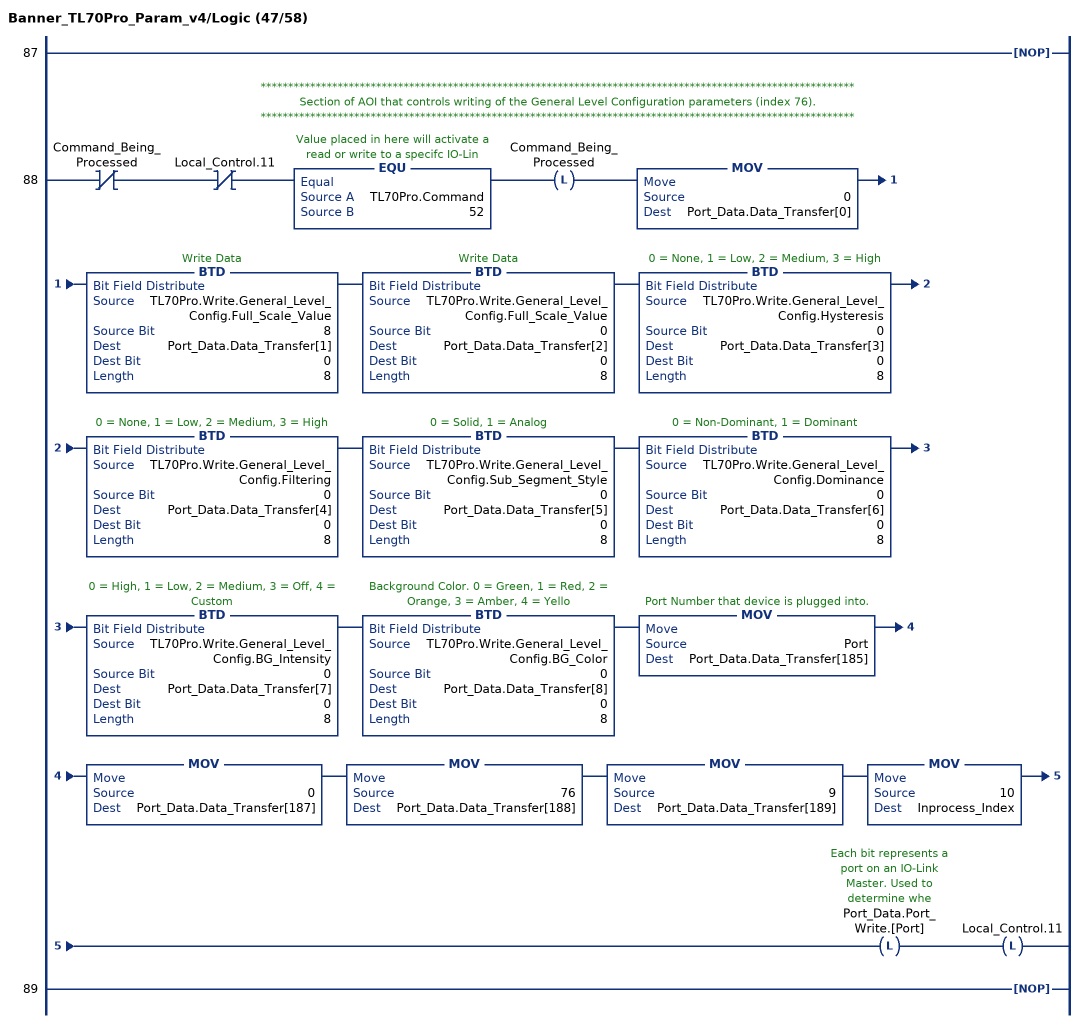
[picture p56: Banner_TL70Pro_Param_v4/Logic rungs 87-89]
   87: NOP();
   // ************************************************************************************************************
   // Section of AOI that controls writing of the General Level Configuration parameters (index 76).
   // ************************************************************************************************************
   88: XIO(Command_Being_Processed)XIO(Local_Control.11)EQU(TL70Pro.Command,52)OTL(Command_Being_Processed)MOV(0,Port_Data.Data_Transfer[0])BTD(TL70Pro.Write.General_Level_Config.Full_Scale_Value,8,Port_Data.Data_Transfer[1],0,8)BTD(TL70Pro.Write.General_Level_Config.Full_Scale_Value,0,Port_Data.Data_Transfer[2],0,8)BTD(TL70Pro.Write.General_Level_Config.Hysteresis,0,Port_Data.Data_Transfer[3],0,8)BTD(TL70Pro.Write.General_Level_Config.Filtering,0,Port_Data.Data_Transfer[4],0,8)BTD(TL70Pro.Write.General_Level_Config.Sub_Segment_Style,0,Port_Data.Data_Transfer[5],0,8)BTD(TL70Pro.Write.General_Level_Config.Dominance,0,Port_Data.Data_Transfer[6],0,8)BTD(TL70Pro.Write.General_Level_Config.BG_Intensity,0,Port_Data.Data_Transfer[7],0,8)BTD(TL70Pro.Write.General_Level_Config.BG_Color,0,Port_Data.Data_Transfer[8],0,8)MOV(Port,Port_Data.Data_Transfer[185])MOV(0,Port_Data.Data_Transfer[187])MOV(76,Port_Data.Data_Transfer[188])MOV(9,Port_Data.Data_Transfer[189])MOV(10,Inprocess_Index)OTL(Port_Data.Port_Write.[Port])OTL(Local_Control.11);
   89: NOP();
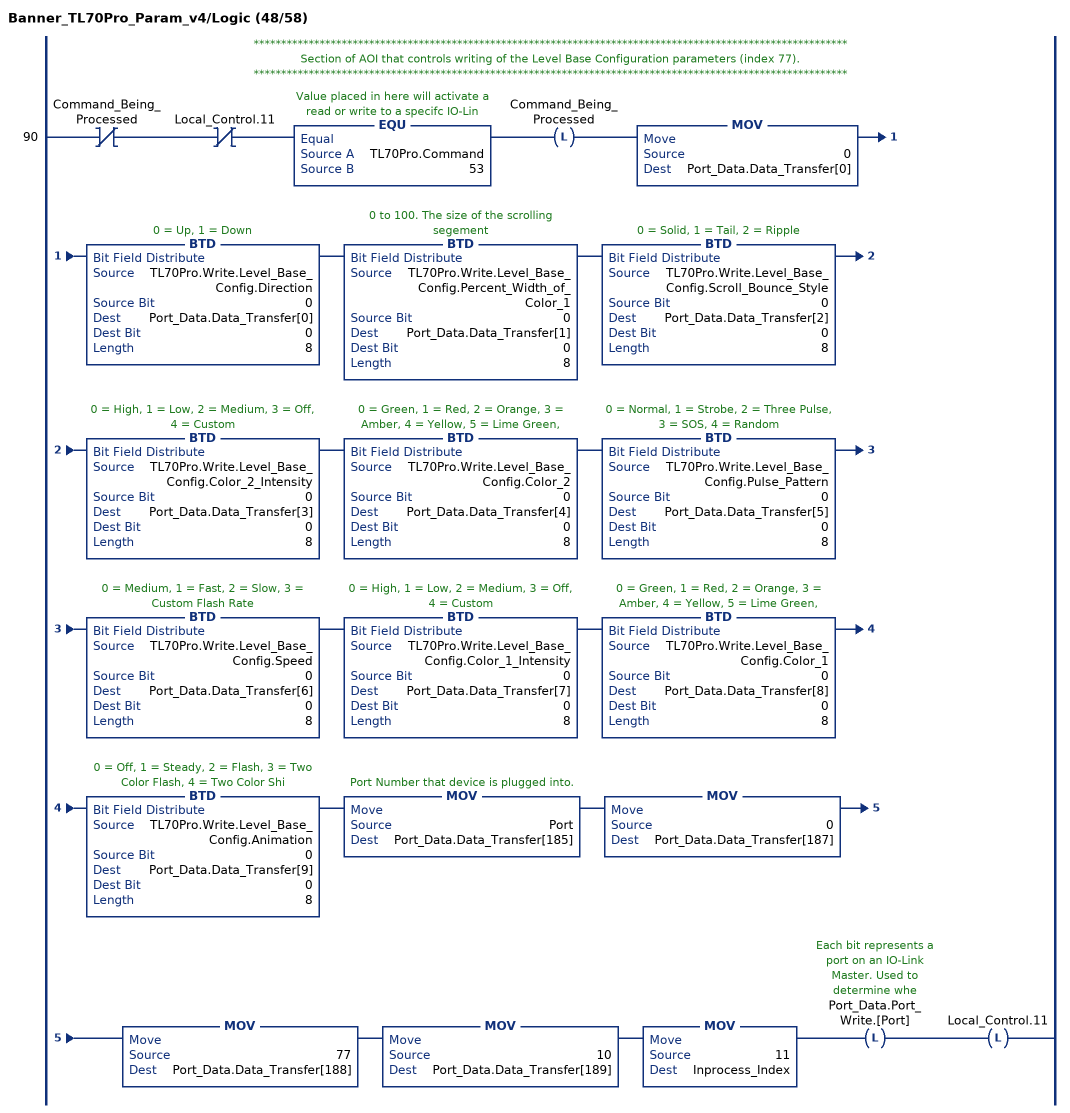
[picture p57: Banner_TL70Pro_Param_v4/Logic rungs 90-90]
   // ************************************************************************************************************
   // Section of AOI that controls writing of the Level Base Configuration parameters (index 77).
   // ************************************************************************************************************
   90: XIO(Command_Being_Processed)XIO(Local_Control.11)EQU(TL70Pro.Command,53)OTL(Command_Being_Processed)MOV(0,Port_Data.Data_Transfer[0])BTD(TL70Pro.Write.Level_Base_Config.Direction,0,Port_Data.Data_Transfer[0],0,8)BTD(TL70Pro.Write.Level_Base_Config.Percent_Width_of_Color_1,0,Port_Data.Data_Transfer[1],0,8)BTD(TL70Pro.Write.Level_Base_Config.Scroll_Bounce_Style,0,Port_Data.Data_Transfer[2],0,8)BTD(TL70Pro.Write.Level_Base_Config.Color_2_Intensity,0,Port_Data.Data_Transfer[3],0,8)BTD(TL70Pro.Write.Level_Base_Config.Color_2,0,Port_Data.Data_Transfer[4],0,8)BTD(TL70Pro.Write.Level_Base_Config.Pulse_Pattern,0,Port_Data.Data_Transfer[5],0,8)BTD(TL70Pro.Write.Level_Base_Config.Speed,0,Port_Data.Data_Transfer[6],0,8)BTD(TL70Pro.Write.Level_Base_Config.Color_1_Intensity,0,Port_Data.Data_Transfer[7],0,8)BTD(TL70Pro.Write.Level_Base_Config.Color_1,0,Port_Data.Data_Transfer[8],0,8)BTD(TL70Pro.Write.Level_Base_Config.Animation,0,Port_Data.Data_Transfer[9],0,8)MOV(Port,Port_Data.Data_Transfer[185])MOV(0,Port_Data.Data_Transfer[187])MOV(77,Port_Data.Data_Transfer[188])MOV(10,Port_Data.Data_Transfer[189])MOV(11,Inprocess_Index)OTL(Port_Data.Port_Write.[Port])OTL(Local_Control.11);
